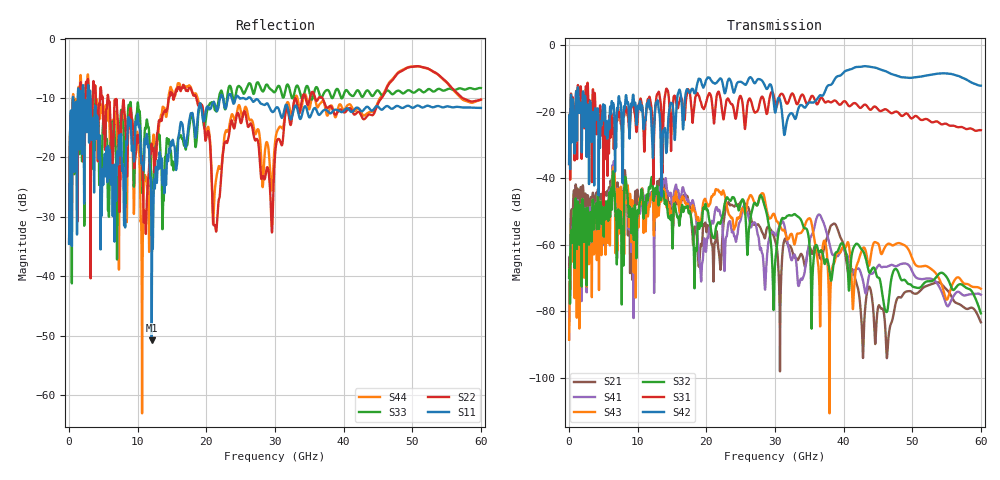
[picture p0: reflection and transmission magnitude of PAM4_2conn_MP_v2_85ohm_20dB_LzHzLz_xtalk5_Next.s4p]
! Info: Touchstone file created by Circ.  Input file=FAB50GbE_2conn_Midplane_Examax_Topo2_v2_85ohm_20dB_LzHzLz.circ
# Hz S RI R 50
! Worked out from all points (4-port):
!   6000 points, 10 MHz to 60 GHz, reference 50 ohm
!   strongest paths, dB at 10 MHz, 15.01 GHz, 30.01 GHz, 45.01 GHz, 60 GHz:
!     S42: -35.6, -17.4, -20.2, -7.0, -12.1
!     S31: -35.8, -20.9, -17.2, -19.2, -25.5
!     S32: -69.9, -55.5, -65.8, -69.8, -80.6
!     S43: -88.6, -51.6, -51.4, -59.6, -73.2
!     S41: -88.2, -48.2, -57.0, -66.3, -75.0
!     S21: -69.5, -51.9, -58.6, -78.9, -83.3
!   lowest |S11| = -50.8 dB at 12.05 GHz (marker M1), VSWR 1.01, Z = 50.3 + j0.115 ohm
!   |S11| at or under -10 dB: 3.115 GHz to 22.02 GHz (18.91 GHz wide, 150 % of centre); 22.42 GHz to 23.15 GHz (730.8 MHz wide, 3.21 % of centre); 26.43 GHz to end of sweep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
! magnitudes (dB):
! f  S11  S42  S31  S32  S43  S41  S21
! 10 MHz  -34.6  -35.6  -35.8  -69.9  -88.6  -88.2  -69.5
! 810 MHz  -18.6  -32.1  -34.6  -65.6  -74.1  -69.3  -52.5
! 6.36 GHz  -29.8  -18.3  -22.0  -39.0  -37.6  -36.0  -37.0
! 12.05 GHz  -50.8  -26.8  -19.9  -39.6  -45.5  -46.2  -44.1
! 22.19 GHz  -9.4  -10.2  -17.8  -52.5  -44.9  -51.3  -63.7
! 38.01 GHz  -12.6  -11.9  -17.1  -68.9  -80.3  -60.3  -54.9
! 60 GHz  -11.7  -12.1  -25.5  -80.6  -73.2  -75.0  -83.3
